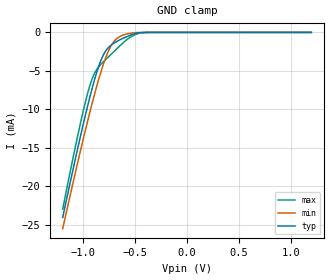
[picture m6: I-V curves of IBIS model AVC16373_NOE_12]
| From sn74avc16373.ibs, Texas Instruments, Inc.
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[Model]   AVC16373_NOE_12
Model_type  Input
Vinl=0
Vinh=1.2
| variable   typ   min   max
C_comp   1.66pF   1.35pF   2.07pF
[Temperature Range]   40   100   -40
| Ambient temperature   25   85   -40
[Voltage range]   1.2   1.2   1.2
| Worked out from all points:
|   GND clamp passes 1 mA (typ) near -0.65 V on its own axis
[GND Clamp]
| AVC16373_NOE_12
|   Voltage   I(typ)   I(min)   I(max)
-1.2V     -24.03mA   -25.47mA   -22.94mA
-1.03V    -13.57mA   -15.44mA   -11.86mA
-970mV    -10.14mA   -12.09mA   -8.455mA
-925mV    -7.733mA   -9.682mA   -6.375mA
-875mV    -5.344mA   -7.158mA   -4.888mA
-840mV    -3.947mA   -5.525mA   -4.273mA
-805mV    -2.871mA   -4.049mA   -3.782mA
-740mV    -1.734mA   -1.915mA   -2.94mA
-675mV    -1.155mA   -772.2uA   -2.095mA
-545mV    -360.3uA   -107.8uA   -609.2uA
-430mV    -20.2uA    -12.29uA   -29.52uA
1.2V      192.9pA    659pA      8.211pA
